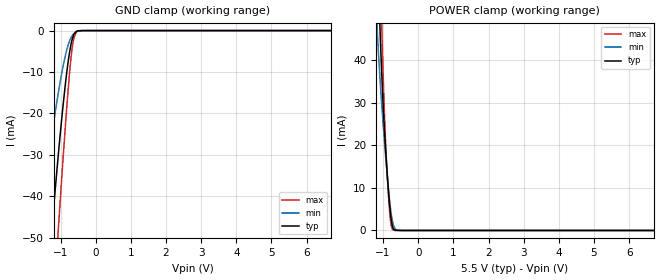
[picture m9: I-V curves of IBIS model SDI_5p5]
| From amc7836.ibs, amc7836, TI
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|   Model
[Model]   SDI_5p5
Model_type   Input
Vinl = 1.65
Vinh = 3.85
|   typ   min   max
C_comp   5.695pF   5.385pF   6.233pF
[Voltage Range]   5.5   5.49   5.51
[Temperature Range]   27   125   -40
[Power Clamp Reference]   5.5   5.49   5.51
[GND Clamp Reference]   0   0   0
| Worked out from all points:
|   GND clamp passes 1 mA (typ) near -0.62 V on its own axis
|   POWER clamp passes 1 mA (typ) near -0.73 V on its own axis
[GND Clamp]
|   Voltage   I(typ)   I(min)   I(max)
-5.5V     -568.4mA   -435.6mA   -672.5mA
-1.595V   -85.95mA   -48.48mA   -120.8mA
-1.26V    -49.31mA   -26.08mA   -74.17mA
-1.111V   -34.46mA   -17.53mA   -54.19mA
-1.062V   -29.78mA   -14.92mA   -47.71mA
-962.5mV  -20.93mA   -10.12mA   -35.09mA
-863.5mV  -12.98mA   -6.046mA   -23.14mA
-781mV    -7.361mA   -3.417mA   -13.98mA
-715mV    -3.861mA   -1.932mA   -7.626mA
-632.5mV  -1.153mA   -826.7uA   -2.253mA
-533.5mV  -131.6uA   -249.6uA   -205.7uA
11V       0A         0A         0A
[POWER Clamp]
|   Voltage   I(typ)   I(min)   I(max)
-5.5V     1.598A     1.344A     1.82A
-1.177V   70.98mA    49.04mA    94.54mA
-1.161V   66.34mA    46.28mA    88.68mA
-1.078V   45.29mA    34.4mA     60.59mA
-1.045V   38.17mA    30.32mA    50.19mA
-1.012V   31.91mA    26.48mA    40.53mA
-946mV    21.55mA    19.33mA    24.41mA
-863.5mV  11.12mA    11.28mA    10.47mA
-781mV    3.338mA    4.739mA    1.874mA
-698.5mV  307.2uA    1.061mA    54.67uA
-484mV    0A         2.951uA    0A
11V       0A         0A         0A
